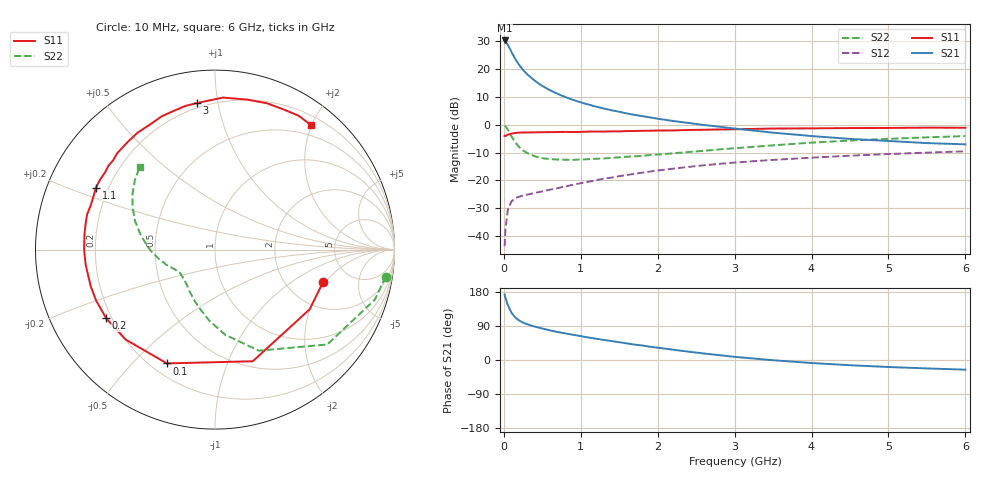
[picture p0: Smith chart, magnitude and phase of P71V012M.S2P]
! SIEMENS Small Signal Semiconductors
! BFP196
! Si NPN RF Bipolar Junction Transistor in SOT143
! VCE = 1 V  IC = 12 mA
! Common Emitter S-Parameters:  May  1996
# GHz  S  MA  R  50
!  f  S11  S21  S12  S22
! GHz  MAG  ANG  MAG  ANG  MAG  ANG  MAG  ANG
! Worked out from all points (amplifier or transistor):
!   36 points, 10 MHz to 6 GHz, reference 50 ohm
!   highest |S21| = 30.1 dB at 10 MHz (marker M1)
!   |S21| within 3 dB of that: start of sweep to 78.42 MHz
!   unconditionally stable (mu >= 1): 797.8 MHz to 5.359 GHz; 5.582 GHz to end of sweep
!   at 250 MHz: K = 0.46, MSG = 22.4 dB, |S12| = -25.4 dB
!   at 1.4 GHz: K = 1.15, MAG = 9.7 dB, |S12| = -19.0 dB
!   at 6 GHz: K = 1.02, MAG = 0.5 dB, |S12| = -9.6 dB
!   S11 on the Smith chart (normalised r, x): 10 MHz: 3.17, -1.89; 100 MHz: 0.26, -0.63; 200 MHz: 0.18, -0.28; 1.1 GHz: 0.15, +0.24; 3 GHz: 0.17, +0.87; 6 GHz: 0.33, +1.99
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0.01  0.6285 -16.7  31.84 173.1  0.0067 83.1  0.9627 -9.0
0.02  0.6237 -32.2  30.75 164.6  0.0128 76.4  0.9331 -17.4
0.05  0.6568 -71.3  26.92 145.6  0.0291 59.5  0.819 -40.2
0.1  0.6884 -112.9  19.7 124.4  0.0427 43.3  0.6135 -66.6
0.15  0.7067 -134.9  14.71 111.9  0.0483 36.5  0.4777 -83.2
0.2  0.717 -147.8  11.62 104.2  0.0514 33.1  0.3957 -94.8
0.25  0.7207 -156.8  9.448 98.6  0.054 32.1  0.3431 -103.7
0.3  0.722 -163.5  7.998 94.5  0.0557 32.3  0.3116 -110.8
0.4  0.7254 -173.3  6.105 88.2  0.0598 33.7  0.2714 -121.6
0.5  0.7294 -179.8  4.896 83.1  0.0639 35.6  0.2504 -129.1
0.6  0.7318 173.9  4.105 78.2  0.0685 37.4  0.2411 -134.6
0.7  0.735 169.0  3.537 73.8  0.073 38.9  0.2367 -139.1
0.8  0.739 164.6  3.095 70.2  0.0784 40.5  0.2353 -142.7
1.1  0.7479 152.5  2.275 59.4  0.0949 43.3  0.2406 -149.5
1.3  0.7487 144.9  1.934 52.9  0.1076 43.7  0.2478 -153.5
1.6  0.7645 135.6  1.577 43.8  0.1255 43.4  0.2657 -158.5
2.2  0.7852 117.5  1.158 27.2  0.1628 39.8  0.3061 -168.1
3  0.8227 97.1  0.848 8.3  0.2093 31.4  0.377 177.2
3.5  0.8482 87.0  0.716 -0.6  0.2336 25.6  0.4252 168.3
4.5  0.8651 70.4  0.554 -13.8  0.2775 14.5  0.5172 152.6
5.5  0.8796 58.0  0.466 -22.2  0.3153 3.5  0.5911 139.0
6  0.8761 52.3  0.443 -25.5  0.3322 -2.4  0.622 132.5
